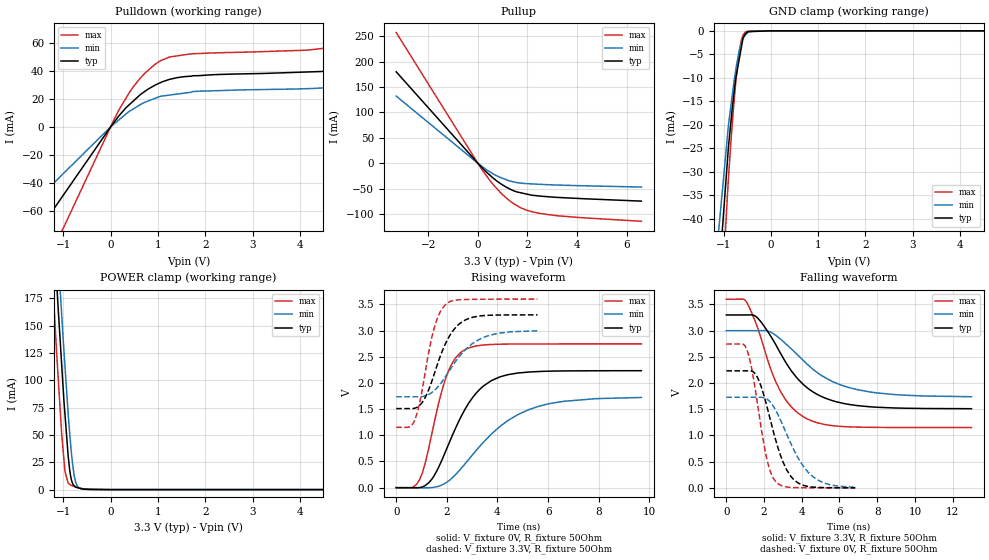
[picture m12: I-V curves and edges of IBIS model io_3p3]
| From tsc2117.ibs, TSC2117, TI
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|   io_3p3 Model
[Model]   io_3p3
Model_type   I/O
Polarity   Non-Inverting
Enable   Active-High
Vinl = 0.99
Vinh = 2.31
Vmeas = 1.65
Vref = 1.65
Cref = 10pF
Rref = 50
|   typ   min   max
|   (nom PVT)   (fast PVT)   (slow PVT)
|C_comp from frequency sweep method (F=14MHz)
|Average
|C_comp   3.200e-12   2.993e-12   3.366e-12
|ON state : BUFFER OUTPUT TURNED HIGH
|C_comp   4.509e-12   4.115e-12   4.826e-12
|OFF state: BUFFER IN HIGH IMPEDANCE
|C_comp   1.891e-12   1.872e-12   1.906e-12
|C_comp from LC tank measurement(L=1nH)
|Average
|Resonant Frequency(Hz)   4.210e+09   4.250e+09   4.170e+09
C_comp   1.439e-12   1.410e-12   1.471e-12
|ON state : BUFFER OUTPUT TURNED HIGH
|Resonant Frequency(Hz)   4.020e+09   4.080e+09   3.950e+09
|C_comp   1.569e-12   1.523e-12   1.625e-12
|OFF state: BUFFER IN HIGH IMPEDANCE
|Resonant Frequency(Hz)   4.400e+09   4.420e+09   4.390e+09
|C_comp   1.310e-12   1.298e-12   1.316e-12
| Where nom  PVT is Nominal Process, 3.3V, 48C
|   Fast PVT is Strong Process,  3.6V, -40C
|   Slow PVT is Weak Process,   3V, 108C
[Model Spec]
|Subparameter   typ   min   max
Vinh   2.31   2.1   2.52
Vinl   0.99   0.9   1.08
[Voltage Range]   3.3   3   3.6
|Ambient Temperature   25   85   -40
|Junction Temperature
[Temperature Range]   48   108   -40
[Pullup Reference]   3.3   3   3.6
[Pulldown Reference]   0   0   0
[Power Clamp Reference]   3.3   3   3.6
[GND Clamp Reference]   0   0   0
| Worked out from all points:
|   slope of the pulldown table from 0 to 0.495 V, typ, clamps not added: 26.1 ohm
|   slope of the pullup table from 0 to 0.495 V, typ, clamps not added: 20.8 ohm
|   GND clamp passes 1 mA (typ) near -0.56 V on its own axis
|   POWER clamp passes 1 mA (typ) near -0.64 V on its own axis
|   falling waveform, V_fixture 3.3V, R_fixture 50Ohm: 20-80 % time 2.17ns typ, 2.72ns min, 1.63ns max; typ from 3.3 V to 1.51 V
|   rising waveform, V_fixture 0V, R_fixture 50Ohm: 20-80 % time 1.4ns typ, 2.22ns min, 854ps max; typ from 0 V to 2.23 V
|   rising waveform, V_fixture 3.3V, R_fixture 50Ohm: 20-80 % time 882ps typ, 1.24ns min, 603ps max; typ from 1.51 V to 3.3 V
|   falling waveform, V_fixture 0V, R_fixture 50Ohm: 20-80 % time 1.09ns typ, 1.46ns min, 765ps max; typ from 2.23 V to 0.001 V
[Pulldown]
|   Voltage   I(typ)   I(min)   I(max)
-3.3V     -161.2mA   -110.2mA   -239mA
-3mV      -146.6uA   -100.2uA   -217.3uA
172.8mV   7.814mA    4.962mA    12.02mA
478.8mV   18.5mA     12.87mA    28.66mA
720mV     25.34mA    17.58mA    38.31mA
1.062V    31.82mA    21.98mA    47.5mA
1.735V    36.63mA    25.3mA     52.44mA
4.162V    39.33mA    27.4mA     54.94mA
4.507V    39.8mA     27.95mA    56.32mA
5.148V    43.41mA    30.52mA    62.67mA
5.67V     50.2mA     35.3mA     74.14mA
6.6V      76.89mA    49.14mA    117.9mA
[GND Clamp]
|   Voltage   I(typ)   I(min)   I(max)
-3.3V     -1.729A    -1.555A    -1.959A
-1.508V   -108.4mA   -86.6mA    -140.4mA
-897.6mV  -24.85mA   -20.19mA   -31.44mA
-788.4mV  -14.1mA    -11.54mA   -16.27mA
-745.8mV  -10.34mA   -8.613mA   -11.35mA
-698.4mV  -7.697mA   -5.818mA   -6.717mA
-622.8mV  -3.48mA    -2.692mA   -1.968mA
-590.7mV  -1.69mA    -1.564mA   -1.022mA
-532.8mV  -607.7uA   -826uA     -209.9uA
-474mV    -183.5uA   -180.3uA   -84.13uA
-285mV    -109.8uA   -1.866uA   -4.827uA
6.6V      0A         0A         0A
[Pullup]
|   Voltage   I(typ)   I(min)   I(max)
-3.3V     180mA      132.2mA    257.1mA
172.8mV   -9.066mA   -6.319mA   -12.96mA
633.6mV   -29.81mA   -21.35mA   -42.9mA
939.6mV   -40.79mA   -28.36mA   -59.08mA
1.246V    -49.52mA   -34.23mA   -72.34mA
1.554V    -56.04mA   -37.69mA   -82.56mA
1.904V    -59.8mA    -39.73mA   -91.02mA
2.473V    -64.21mA   -41.21mA   -98.18mA
4.162V    -69.36mA   -44.01mA   -106.8mA
6.6V      -74.32mA   -46.7mA    -114mA
[POWER Clamp]
|   Voltage   I(typ)   I(min)   I(max)
-3.3V     1.958A     1.976A     1.945A
-1.339V   341.9mA    389.7mA    280.9mA
-1.156V   201.8mA    248.4mA    136.7mA
-1.134V   185.3mA    231.8mA    120.6mA
-1.115V   171.1mA    218.5mA    107.6mA
-1.037V   116.3mA    162.4mA    52.94mA
-964.8mV  69.07mA    113.3mA    16.78mA
-897.6mV  31.05mA    70.07mA    6.041mA
-828mV    8.841mA    33.42mA    3.831mA
-741mV    2.422mA    7.23mA     2.378mA
-591mV    617.8uA    482.1uA    906.8uA
6.6V      0A         0A         0A
[Ramp]
R_load = 50
|   typ   min   max
dV/dt_r   1.34026/1.39657e-09   1.03733/2.23289e-09   1.64702/8.49823e-10
dV/dt_f   1.07345/2.17251e-09   0.756216/2.71558e-09   1.46866/1.62606e-09
[Falling Waveform]
V_fixture = 3.3V
V_fixture_min = 3V
V_fixture_max = 3.6V
R_fixture = 50Ohm
|   Time   V(typ)   V(min)   V(max)
0s        3.3V       3V         3.6V
1.057ns   3.3V       3V         3.554V
1.661ns   3.241V     3V         3.054V
2.336ns   2.905V     2.974V     2.285V
2.787ns   2.624V     2.865V     1.9V
3.446ns   2.234V     2.653V     1.547V
4.236ns   1.926V     2.378V     1.326V
5.313ns   1.703V     2.088V     1.204V
6.945ns   1.57V      1.875V     1.16V
13ns      1.511V     1.74V      1.152V
[Rising Waveform]
V_fixture = 0V
V_fixture_min = 0V
V_fixture_max = 0V
R_fixture = 50Ohm
|   Time   V(typ)   V(min)   V(max)
0s        2.397nV    8.663nV    828.8pV
643ps     -756.2uV   -4.801uV   3.928mV
921ps     690.6uV    -313.1uV   155.2mV
1.135ns   37.58mV    -2.285mV   447.9mV
1.412ns   166.2mV    1.389mV    1.043V
1.987ns   735.7mV    100.2mV    2.132V
2.685ns   1.468V     435.9mV    2.625V
3.746ns   2.04V      1.017V     2.734V
5.239ns   2.208V     1.49V      2.744V
9.683ns   2.233V     1.722V     2.745V
[Rising Waveform]
V_fixture = 3.3V
V_fixture_min = 3V
V_fixture_max = 3.6V
R_fixture = 50Ohm
|   Time   V(typ)   V(min)   V(max)
0s        1.51V      1.735V     1.152V
514ps     1.51V      1.735V     1.159V
731ps     1.517V     1.735V     1.291V
933ps     1.575V     1.735V     1.635V
1.124ns   1.704V     1.749V     2.14V
1.474ns   2.128V     1.843V     3.002V
1.98ns    2.784V     2.145V     3.51V
2.607ns   3.168V     2.57V      3.591V
3.322ns   3.279V     2.841V     3.597V
5.58ns    3.299V     2.995V     3.6V
[Falling Waveform]
V_fixture = 0V
V_fixture_min = 0V
V_fixture_max = 0V
R_fixture = 50Ohm
|   Time   V(typ)   V(min)   V(max)
0s        2.234V     1.73V      2.745V
1.089ns   2.234V     1.73V      2.637V
1.373ns   2.226V     1.73V      2.221V
1.739ns   2.038V     1.73V      1.399V
2.175ns   1.522V     1.691V     511.3mV
2.616ns   915.2mV    1.481V     120.6mV
3.402ns   229.1mV    861.7mV    8.733mV
4.361ns   24.84mV    290.1mV    1.778mV
5.203ns   5.198mV    90.73mV    890.2uV
6.836ns   1.043mV    9.752mV    279.2uV
